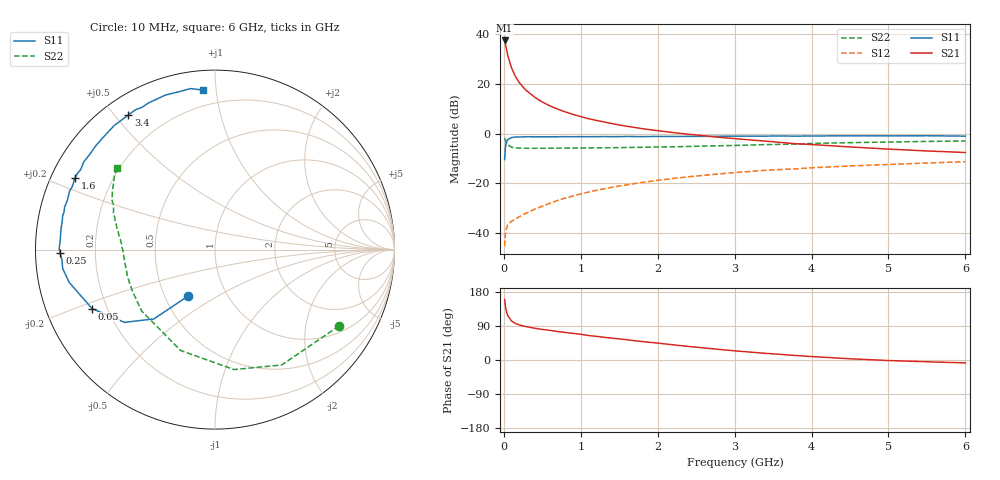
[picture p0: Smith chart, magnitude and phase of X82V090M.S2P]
! SIEMENS Small Signal Semiconductors
! BFP136W
! Si NPN RF Bipolar Junction Transistor in SOT343
! VCE = 2 V  IC = 90 mA
! Common Emitter S-Parameters:  September  1994
# GHz  S  MA  R  50
!  f  S11  S21  S12  S22
! GHz  MAG  ANG  MAG  ANG  MAG  ANG  MAG  ANG
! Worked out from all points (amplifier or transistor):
!   40 points, 10 MHz to 6 GHz, reference 50 ohm
!   highest |S21| = 37.6 dB at 10 MHz (marker M1)
!   |S21| within 3 dB of that: start of sweep to 30.64 MHz
!   unconditionally stable (mu >= 1): 472.8 MHz to 2.884 GHz
!   at 200 MHz: K = 0.70, MSG = 27.1 dB, |S12| = -33.5 dB
!   at 1.5 GHz: K = 1.11, MAG = 10.3 dB, |S12| = -21.1 dB
!   at 6 GHz: K = 0.98, MSG = 1.9 dB, |S12| = -11.3 dB
!   S11 on the Smith chart (normalised r, x): 10 MHz: 0.65, -0.37; 50 MHz: 0.14, -0.22; 250 MHz: 0.07, -0.01; 1.6 GHz: 0.07, +0.24; 3.4 GHz: 0.07, +0.54; 6 GHz: 0.11, +0.92
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0.01  0.3012 -120.3  75.52 159.7  0.0054 69.8  0.8119 -31.6
0.02  0.5149 -131.4  64.41 143.0  0.0096 55.5  0.7425 -60.0
0.03  0.6469 -141.2  54.06 131.2  0.0119 48.2  0.6767 -81.0
0.05  0.7599 -154.4  38.29 117.2  0.0145 38.0  0.5938 -108.8
0.1  0.8325 -167.3  21.06 102.9  0.0172 36.0  0.5329 -140.0
0.15  0.8551 -172.9  14.31 96.6  0.0189 38.4  0.5155 -152.7
0.2  0.8547 -176.0  10.73 92.7  0.0211 41.7  0.5108 -159.6
0.25  0.8623 -178.6  8.65 89.9  0.0233 45.0  0.5092 -164.0
0.3  0.8682 179.6  7.231 87.7  0.0253 48.1  0.5067 -166.9
0.4  0.8635 176.3  5.442 83.9  0.03 53.3  0.5072 -170.8
0.5  0.8652 173.6  4.343 80.7  0.0345 56.1  0.5078 -173.5
0.6  0.8655 171.8  3.622 78.2  0.0397 58.0  0.5085 -175.2
0.7  0.8656 169.3  3.122 75.1  0.0451 60.4  0.5099 -176.5
0.9  0.8669 165.9  2.444 70.1  0.0555 61.5  0.5122 -179.0
1.1  0.8672 161.5  2.001 64.6  0.0664 61.9  0.516 179.4
1.6  0.877 153.0  1.407 53.5  0.093 60.3  0.5261 175.4
2.2  0.8768 142.8  1.052 40.1  0.1248 55.7  0.5433 170.8
3.2  0.89 125.8  0.747 20.9  0.1729 46.1  0.5884 161.9
3.4  0.892 122.8  0.707 17.6  0.1825 43.8  0.6016 160.1
4.5  0.9044 107.7  0.54 3.2  0.2229 33.4  0.6592 150.2
5.5  0.9074 98.6  0.448 -4.7  0.2558 25.4  0.6973 143.4
6  0.8912 94.4  0.417 -7.7  0.272 21.0  0.7118 140.4
